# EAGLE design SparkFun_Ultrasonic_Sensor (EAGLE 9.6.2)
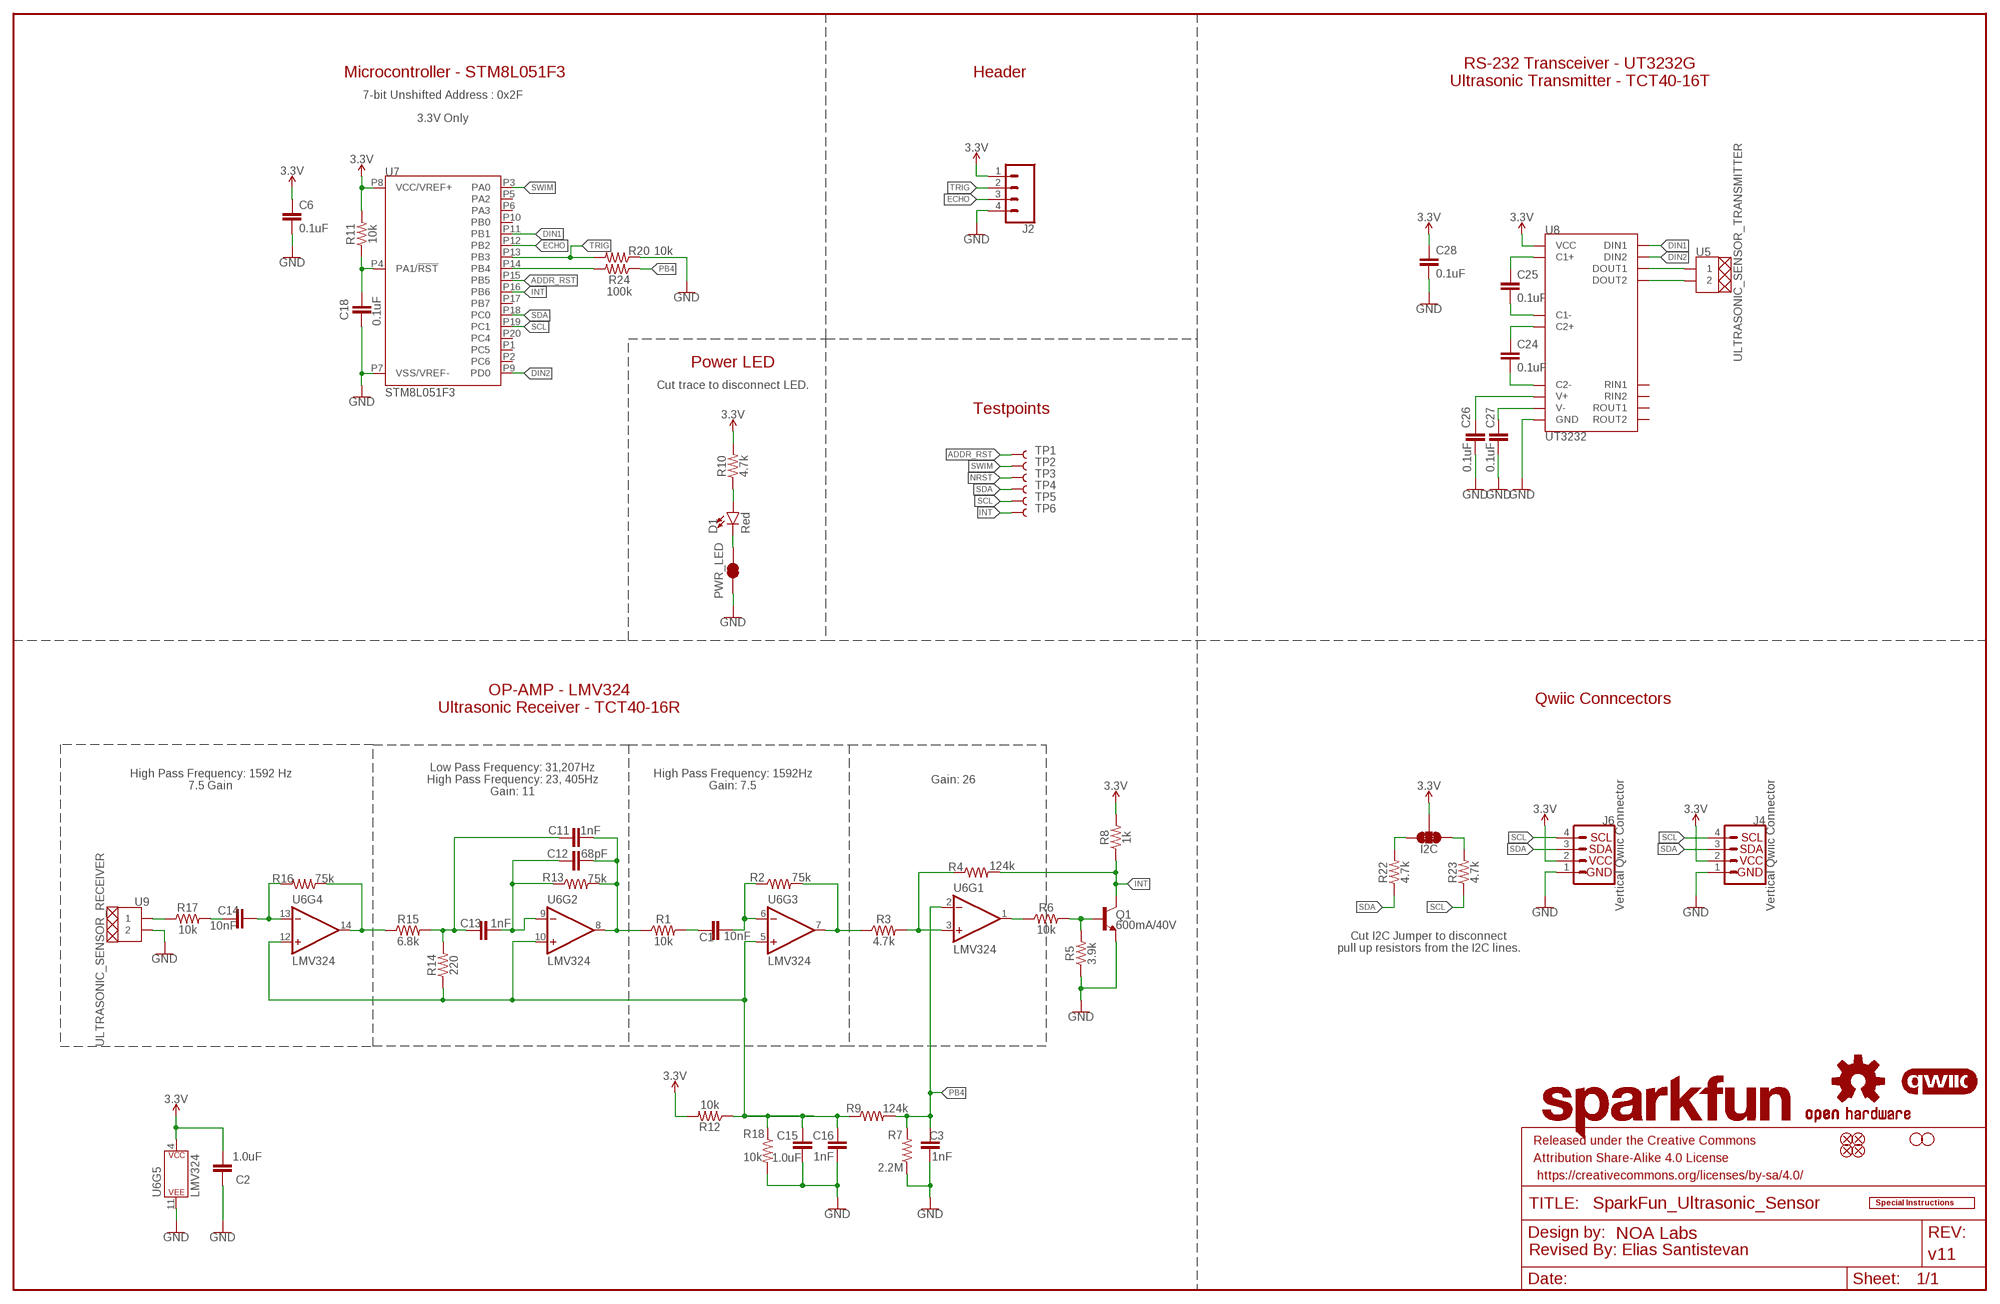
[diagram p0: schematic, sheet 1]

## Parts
C1  10nF  10NF-0603-50V-10%  [0603]
C2  1.0uF  1.0UF-0603-16V-10%  [0603]
C3  1nF  1.0NF/1000PF-0603-50V-10%  [0603]
C6  0.1uF  0.1UF-0603-25V-(+80/-20%)  [0603]
C11  1nF  1.0NF/1000PF-0603-50V-10%  [0603]
C12  68pF  68PF-0603-50V-5%  [0603]
C13  1nF  1.0NF/1000PF-0603-50V-10%  [0603]
C14  10nF  10NF-0603-50V-10%  [0603]
C15  1.0uF  1.0UF-0603-16V-10%  [0603]
C16  1nF  1.0NF/1000PF-0603-50V-10%  [0603]
C18  0.1uF  0.1UF-0603-25V-(+80/-20%)  [0603]
C24  0.1uF  0.1UF-0603-25V-(+80/-20%)  [0603]
C25  0.1uF  0.1UF-0603-25V-(+80/-20%)  [0603]
C26  0.1uF  0.1UF-0603-25V-(+80/-20%)  [0603]
C27  0.1uF  0.1UF-0603-25V-(+80/-20%)  [0603]
C28  0.1uF  0.1UF-0603-25V-(+80/-20%)  [0603]
D1  Red  LED-RED_0603-KB  [LED-0603]
FD1  FIDUCIAL1X2  [FIDUCIAL-1X2]
FD2  FIDUCIAL1X2  [FIDUCIAL-1X2]
FD3  FIDUCIAL1X2  [FIDUCIAL-1X2]
FD4  FIDUCIAL1X2  [FIDUCIAL-1X2]
FRAME1  FRAME-LEDGER  [CREATIVE_COMMONS]
H1  STAND-OFFTIGHT  [STAND-OFF-TIGHT]
H2  STAND-OFFTIGHT  [STAND-OFF-TIGHT]
I2C  JUMPER-SMT_3_2-NC_TRACE_SILK  [SMT-JUMPER_3_2-NC_TRACE_SILK]
J2  CONN_041X04_NO_SILK_NO_POP  [1X04_NO_SILK]
J4  Vertical Qwiic Connector  QWIIC_CONNECTOR  [JST04_1MM_VERT]
J6  Vertical Qwiic Connector  QWIIC_CONNECTOR  [JST04_1MM_VERT]
LOGO1  SPECIAL_INSTRUCTIONS-ORDERING  [ORDERING_INSTRUCTIONS]
LOGO2  SFE_LOGO_NAME.1_INCH  [SFE_LOGO_NAME_.1]
LOGO3  QWIIC_LOGO_3MM  [QWIIC_3MM]
LOGO4  OSHW-LOGOS  [OSHW-LOGO-S]
PWR_LED  JUMPER-SMT_2_NC_TRACE_SILK  [SMT-JUMPER_2_NC_TRACE_SILK]
Q1  600mA/40V  TRANS_NPN-MMBT2222AL  [SOT23-3]
R1  10k  10KOHM-0603-1/10W-1%  [0603]
R2  75k  75KOHM-0603-1/10W-1%  [0603]
R3  4.7k  4.7KOHM-0603-1/10W-1%  [0603]
R4  124k  124KOHM  [0603]
R5  3.9k  3.9KOHM-0603-1/10W-1%  [0603]
R6  10k  10KOHM-0603-1/10W-1%  [0603]
R7  2.2M  2.2MOHMS-0603-1/10W-1%  [0603]
R8  1k  1KOHM-0603-1/10W-1%  [0603]
R9  124k  124KOHM  [0603]
R10  4.7k  4.7KOHM-0603-1/10W-1%  [0603]
R11  10k  10KOHM-0603-1/10W-1%  [0603]
R12  10k  10KOHM-0603-1/10W-1%  [0603]
R13  75k  75KOHM-0603-1/10W-1%  [0603]
R14  220  220OHM-0603-1/10W-1%  [0603]
R15  6.8k  6.8KOHM-0603-1/10W-1%  [0603]
R16  75k  75KOHM-0603-1/10W-1%  [0603]
R17  10k  10KOHM-0603-1/10W-1%  [0603]
R18  10k  10KOHM-0603-1/10W-1%  [0603]
R20  10k  10KOHM-0603-1/10W-1%  [0603]
R22  4.7k  4.7KOHM-0603-1/10W-1%  [0603]
R23  4.7k  4.7KOHM-0603-1/10W-1%  [0603]
R24  100k  100KOHM-0603-1/10W-1%  [0603]
TP1  TEST-POINT3X5  [PAD.03X.05]
TP2  TEST-POINT3X5  [PAD.03X.05]
TP3  TEST-POINT3X5  [PAD.03X.05]
TP4  TEST-POINT3X5  [PAD.03X.05]
TP5  TEST-POINT3X5  [PAD.03X.05]
TP6  TEST-POINT3X5  [PAD.03X.05]
U5  ULTRASONIC_SENSOR_TRANSMITTER  [TFT40-16T]
U6  LMV324  [SO14]
U7  STM8L051F3  [TSSOP20]
U8  UT3232  [TSSOP16]
U9  ULTRASONIC_SENSOR_RECEIVER  [TCT40-16R]

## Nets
3.3V: C2.2 C6.1 C28.1 I2C.2 J2.1 J4.2 J6.2 R8.2 R10.2 R11.2 R12.2 U6.4(P$V+) U7.P8(VCC/VREF+) U8.P16(VCC)
ADDR_RST: TP1.1 U7.P15(PB5)
DIN1: U7.P11(PB1) U8.P11(DIN1)
DIN2: U7.P9(PD0) U8.P10(DIN2)
ECHO: J2.3 U7.P12(PB2)
GND: C2.1 C3.2 C6.2 C15.1 C16.1 C18.2 C26.2 C27.2 C28.2 J2.4 J4.1 J6.1 PWR_LED.1 Q1.2(E) R5.1 R7.1 R18.2 R20.1 U6.11(P$V-) U7.P7(VSS/VREF-) U8.P15(GND) U9.P2
INT: Q1.3(C) R4.2 R8.1 TP6.1 U7.P16(PB6)
N: R24.2 U7.P14(PB4)
N$1: R2.2 R3.1 U6.7(OUT)
N$2: C1.1 R2.1 U6.6(-IN)
N$3: C1.2 R1.2
N$4: R3.2 R4.1 U6.3(+IN)
N$5: Q1.1(B) R5.2 R6.2
N$6: R6.1 U6.1(OUT)
N$7: D1.A R10.1
N$8: C25.1 U8.P1(C1+)
N$9: C12.1 C13.1 R13.1 U6.9(-IN)
N$10: C11.2 C12.2 R1.1 R13.2 U6.8(OUT)
N$11: D1.C PWR_LED.2
N$12: C11.1 C13.2 R14.2 R15.2
N$14: R15.1 R16.1 U6.14(OUT)
N$15: C14.1 R16.2 U6.13(-IN)
N$16: C14.2 R17.2
N$19: I2C.3 R22.2
N$20: I2C.1 R23.2
N$26: R17.1 U9.P1
N$31: C15.2 C16.2 R9.1 R12.1 R14.1 R18.1 U6.5(+IN) U6.10(+IN) U6.12(+IN)
N$37: C25.2 U8.P3(C1-)
N$38: C24.1 U8.P4(C2+)
N$39: C24.2 U8.P5(C2-)
N$40: C27.1 U8.P6(V-)
N$41: C26.1 U8.P2(V+)
N$48: U5.P1 U8.P14(DOUT1)
N$49: U5.P2 U8.P7(DOUT2)
NRST: C18.1 R11.1 TP3.1 U7.P4(PA1/!RST!)
PB4: C3.1 R7.2 R9.2 R24.1 U6.2(-IN)
SCL: J4.4 J6.4 R23.1 TP5.1 U7.P19(PC1)
SDA: J4.3 J6.3 R22.1 TP4.1 U7.P18(PC0)
SWIM: TP2.1 U7.P3(PA0)
TRIG: J2.2 R20.2 U7.P13(PB3)
Unconnected: U7.P1(PC5) U7.P2(PC6) U7.P5(PA2) U7.P6(PA3) U7.P10(PB0) U7.P17(PB7) U7.P20(PC4) U8.P8(RIN2) U8.P9(ROUT2) U8.P12(ROUT1) U8.P13(RIN1)

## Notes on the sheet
- Microcontroller - STM8L051F3 | Header
- RS-232 Transceiver - UT3232G
  Ultrasonic Transmitter - TCT40-16T
- 7-bit Unshifted Address : 0x2F
- 3.3V Only
- Power LED
- Cut trace to disconnect LED.
- Testpoints
- OP-AMP - LMV324
  Ultrasonic Receiver - TCT40-16R
- Qwiic Conncectors
- High Pass Frequency: 1592 Hz
  7.5 Gain
- Low Pass Frequency: 31,207Hz
  High Pass Frequency: 23, 405Hz
  Gain: 11
- High Pass Frequency: 1592Hz
  Gain: 7.5
- Gain: 26
- Cut I2C Jumper to disconnect
  pull up resistors from the I2C lines.
- Revised By: Elias Santistevan

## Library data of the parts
C1 C14 = SparkFun-Capacitors:10NF: 0.01uF/10nF/10,000pF ceramic capacitors; PROD_ID: CAP-00867
C2 C15 = SparkFun-Capacitors:1.0UF: 1µF ceramic capacitors; PROD_ID: CAP-00868
C3 C11 C13 C16 = SparkFun-Capacitors:1.0NF/1000PF: 1nF/1,000pF ceramic capacitors; PROD_ID: CAP-07886
C6 C18 C24-C28 = SparkFun-Capacitors:0.1UF: 0.1µF ceramic capacitors; PROD_ID: CAP-00810
C12 = SparkFun-Capacitors:68PF: 68pF ceramic capacitors; PROD_ID: CAP-14092
D1 = SparkFun-LED:LED-RED: Red SMD LED; PROD_ID: DIO-17976
FD1-FD4 = SparkFun-Aesthetics:FIDUCIAL: Fiducial Alignment Points
FRAME1 = SparkFun-Aesthetics:FRAME-LEDGER: Schematic Frame - Ledger; DESIGNER: NOA Labs; REV: v11
H1 H2 = SparkFun-Hardware:STAND-OFF: Stand Off
I2C = SparkFun-Jumpers:JUMPER-SMT_3_2-NC_TRACE: Normally closed trace jumper (2 of 2 connections) This jumper has a trace between all three pads so they are normally closed (NC). Use a razor knife to open the connection(s). For best results follow the IPC guidelines for cutting traces: Cutout at least 0.063 mm (0.005 in). Remove all loose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
J2 = SparkFun-Connectors:CONN_04: Multi connection point. Often used as Generic Header-pin footprint for 0.1 inch spaced/style header connections On any of the 0.1 inch spaced packages, you can populate with these: Break Away Headers - Straight (PRT-00116) Break Away Male Headers - Right Angle (PRT-00553) Female Headers (PRT-00115)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
J4 J6 = SparkFun-Connectors:QWIIC_CONNECTOR: SparkFun I2C Standard Qwiic Connector An SMD 1mm pitch JST connector makes it easy and quick (get it? Qwiic?) to connect I2C devices to each other. The Qwiic system enables fast and solderless connection between popular platforms and various sensors and actuators. We carry 200mm, 100mm, 50mm, and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; PROD_ID: CONN-14483
LOGO1 = SparkFun-Aesthetics:SPECIAL_INSTRUCTIONS: Special Ordering/Production Instructions Alert
LOGO2 = SparkFun-Aesthetics:SFE_LOGO_NAME: SparkFun Font Logo
LOGO3 = SparkFun-Aesthetics:QWIIC_LOGO: Qwiic Logos for placement on schematic and PCB. The 5.5mm silk logo is best for placing next to Qwiic connector.
LOGO4 = SparkFun-Aesthetics:OSHW-LOGO: Open-Source Hardware (OSHW) Logo
PWR_LED = SparkFun-Jumpers:JUMPER-SMT_2_NC_TRACE: Normally closed trace jumper
Q1 = SparkFun-DiscreteSemi:TRANS_NPN: NPN transistor Current controlled devices typically used to amplify current or used as a switch. BC547 - COM-08928 (TO-92 45V 100mA) (1.Collector 2.Base 3.Emitter) 2N3904 - COM-00521 (TO-92 40V 200mA) (1.Emitter 2.Base 3.Collector) P2N2222A - COM-12852 (TO-92 40V 600mA) (1.Collector 2.Base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; PROD_ID: TRANS-08049
R1 R6 R11 R12 R17 R18 R20 = SparkFun-Resistors:10KOHM: 10kΩ resistor; PROD_ID: RES-00824
R2 R13 R16 = SparkFun-Resistors:75KOHM: 75kΩ resistor; PROD_ID: RES-09737
R3 R10 R22 R23 = SparkFun-Resistors:4.7KOHM: 4.7kΩ resistor; PROD_ID: RES-07857
R4 R9 = SparkFun-Resistors:124KOHM: 124kΩ resistor; PROD_ID: RES-14395
R5 = SparkFun-Resistors:3.9KOHM: 3.9kΩ resistor; PROD_ID: RES-08701
R7 = SparkFun-Resistors:2.2MOHMS: 2MΩ resistor; PROD_ID: RES-10054
R8 = SparkFun-Resistors:1KOHM: 1kΩ resistor; PROD_ID: RES-07856
R14 = SparkFun-Resistors:220OHM: 220Ω resistor; PROD_ID: RES-07861
R15 = SparkFun-Resistors:6.8KOHM: 6.8kΩ resistor; PROD_ID: RES-08597
R24 = SparkFun-Resistors:100KOHM: 100kΩ resistor; PROD_ID: RES-07828
TP1-TP6 = SparkFun-Connectors:TEST-POINT: SparkFun Test Points
U5 = new_parts:ULTRASONIC_SENSOR: CU Devices - CUSA-R/T80; PROD_ID: SEN-21316
U6 = SparkFun-IC-Amplifiers:LMV324: IC LMV324 Quad Op Amp Jellybean quad op-amp Datasheet SparkFun Products SparkFun Sensor Kit (DEV-13754) SparkFun Inventor's Kit for Arduino 101 (KIT-13844) SparkFun Sound Detector (SEN-12642); PROD_ID: IC-08227
U7 = new_parts:STM8L051F3: ST STM8L051F3 Low-Power MCU STM8L051F3 features an enhanced STM8 CPU core providing increased processing power (up to 16 MIPS at 16 MHz) while maintaining the advantages of a CISC architecture with improved code density, a 24-bit linear addressing space and an optimized architecture for low-power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; PROD_ID: IC-21318
U8 = new_parts:UT3232: Unisonic Technologies - UT3232 TThe UTC UT3232 has two receivers and two drivers, and a dual charge-pump circuit. The device meets the requirements of TIA/EIA-232-F and provides the electrical interface between an asynchronous communication controller and the serial-port connector. The charge pump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; PROD_ID: IC-21317
U9 = new_parts:ULTRASONIC_SENSOR: CU Devices - CUSA-R/T80; PROD_ID: SEN-21315

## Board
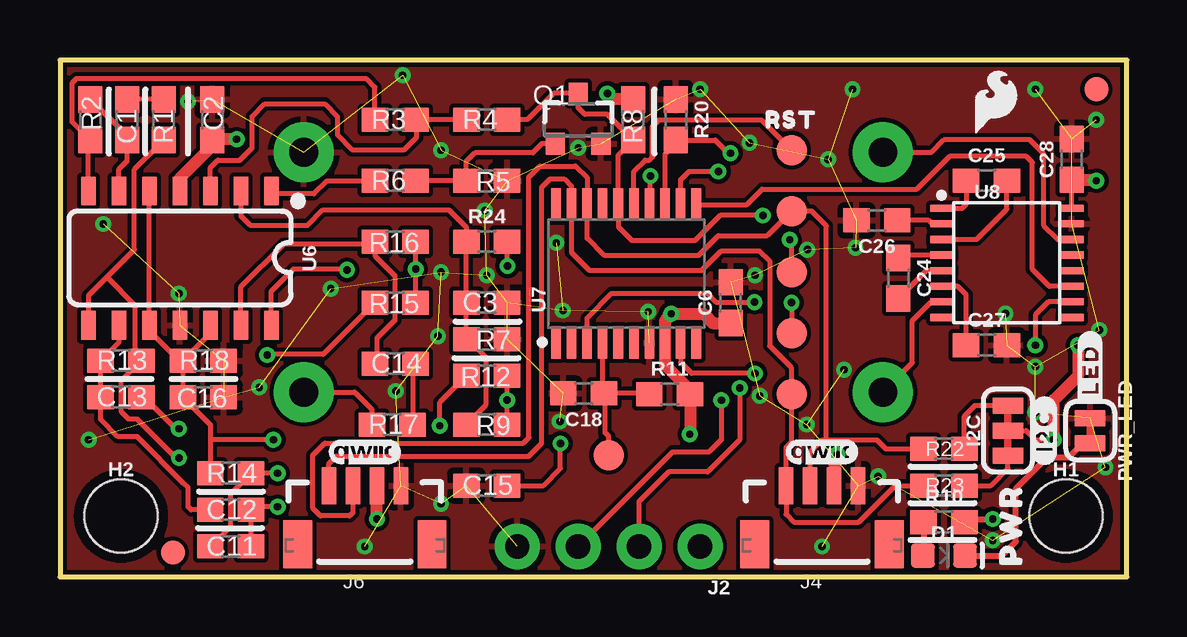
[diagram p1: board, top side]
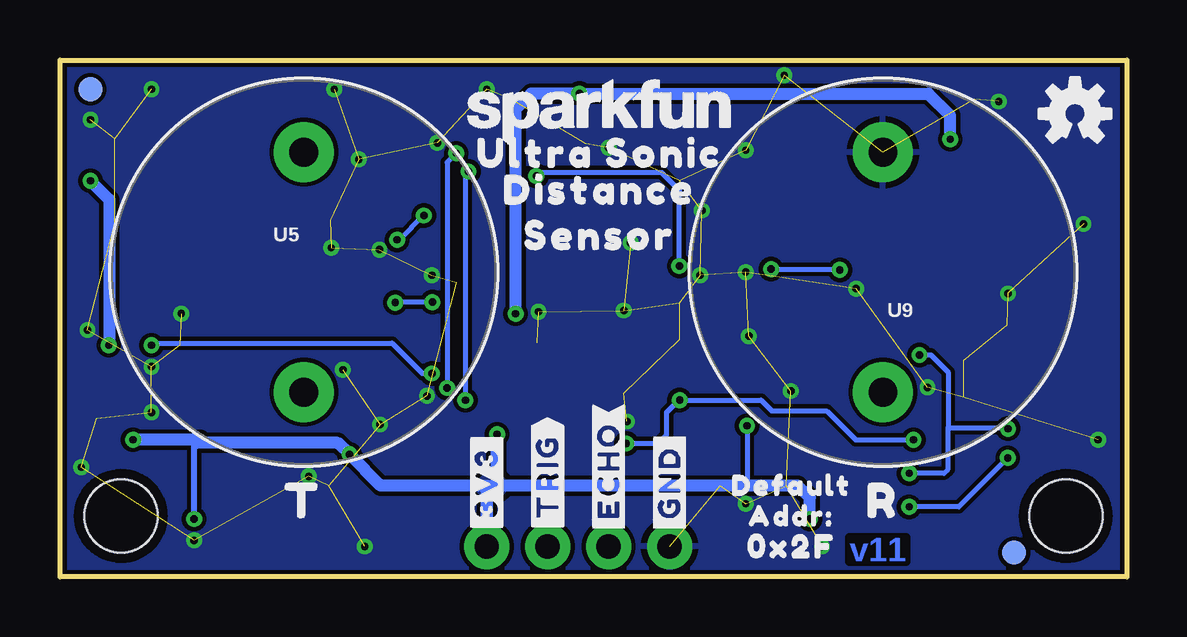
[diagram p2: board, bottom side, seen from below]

Size 44.45 x 21.54 mm. Coordinates in mm from the lower left corner, seen from the top.
Outline: 0,0 44.45,0 44.45,21.54 0,21.54 0,0
Copper layers (1+16): Top 0.035559375mm / dielectric 0.47751875mm / Bottom 0.035559375mm
Design rules "SparkFun-4-Layer-General-JLCPCB *": minimum track width 7mil, minimum drill 12mil, track to track 7mil, track to pad 7mil, pad to pad 7mil, via to via 7mil, smd to smd 7mil, copper to edge 7mil, drill to drill 7mil, minimum pad ring 7mil, minimum via ring 7mil, stop-mask expansion 3mil, vias tented up to drill 25mil, thermal gap 10mil

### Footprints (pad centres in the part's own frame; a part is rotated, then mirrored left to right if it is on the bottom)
0603 = smd 1.1 x 1: 1 -0.85,0; 2 0.85,0
LED-0603 = smd 1 x 1: A -0.877,0; C 0.877,0
FIDUCIAL-1X2 = smd 1 x 1: 1 0,0
STAND-OFF-TIGHT = hole 3.048: 0,0
SMT-JUMPER_3_2-NC_TRACE_SILK = smd 0.66 x 1.27: 1 -1.041,0; 2 0,0; 3 1.041,0
1X04_NO_SILK = drill 1.016 pad 1.88: 1 0,0; 2 2.54,0; 3 5.08,0; 4 7.62,0
JST04_1MM_VERT = smd 0.6 x 1.55: 1 -1.5,0.775; 2 -0.5,0.775; 3 0.5,0.775; 4 1.5,0.775 | smd 1.2 x 2: NC1 -2.8,3.2; NC2 2.8,3.2
SMT-JUMPER_2_NC_TRACE_SILK = smd 0.66 x 1.27: 1 -0.521,0; 2 0.521,0
SOT23-3 = smd 0.8 x 0.9: 1 -0.95,-1; 2 0.95,-1; 3 0,1.1
PAD.03X.05 = smd 1.27 x 1.27: 1 0,0
TFT40-16T = drill 1.2 pad 2.5: P1 0,5; P2 0,-5
SO14 = smd 0.6 x 1.2: 1 -3.175,-2.8; 2 -1.905,-2.8; 3 -0.635,-2.8; 4 0.635,-2.8; 5 1.905,-2.8; 6 3.175,-2.8; 7 4.445,-2.8; 8 4.445,2.8; 9 3.175,2.8; 10 1.905,2.8; 11 0.635,2.8; 12 -0.635,2.8; 13 -1.905,2.8; 14 -3.175,2.8
TSSOP20 = smd 1.35 x 0.4: P1 -2.911,2.878; P2 -2.911,2.228; P3 -2.911,1.578; P4 -2.911,0.928; P5 -2.911,0.278; P6 -2.911,-0.372; P7 -2.911,-1.022; P8 -2.911,-1.672; P9 -2.911,-2.322; P10 -2.911,-2.972; P11 2.839,-2.972; P12 2.839,-2.322; P13 2.839,-1.672; P14 2.839,-1.022; P15 2.839,-0.372; P16 2.839,0.278; P17 2.839,0.928; P18 2.839,1.578; P19 2.839,2.228; P20 2.839,2.878
TSSOP16 = smd 1 x 0.3: P1 -2.607,2.153; P2 -2.607,1.503; P3 -2.607,0.853; P4 -2.607,0.203; P5 -2.607,-0.447; P6 -2.607,-1.097; P7 -2.607,-1.747; P8 -2.607,-2.397; P9 2.793,-2.397; P10 2.793,-1.747; P11 2.793,-1.097; P12 2.793,-0.447; P13 2.793,0.203; P14 2.793,0.853; P15 2.793,1.503; P16 2.793,2.153
TCT40-16R = drill 1.2 pad 2.5: P1 0,5; P2 0,-5

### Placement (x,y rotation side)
C1  2.79,19.05 90 top
C2  6.35,19.05 270 top
C3  17.78,11.43 0 top
C6  27.94,11.43 90 top
C11  7.11,1.27 0 top
C12  7.11,2.79 0 top
C13  2.54,7.49 0 top
C14  13.97,8.89 0 top
C15  17.78,3.81 0 top
C16  5.97,7.49 180 top
C18  21.82,7.65 180 top
C24  34.92,12.45 270 top
C25  38.61,16.51 0 top
C26  34.04,14.86 180 top
C27  38.61,9.65 0 top
C28  42.16,17.4 90 top
D1  36.83,0.89 0 top
FD1  4.7,1.02 90 top
FD2  43.18,20.32 90 top
FD3  43.18,20.32 90 bottom
FD4  4.7,1.02 90 bottom
FRAME1  not placed on the board
H1  41.91,2.54 0 top
H2  2.54,2.54 0 top
I2C  39.5,6.1 90 top
J2  26.67,1.27 180 top
J4  31.75,4.57 180 top
J6  12.7,4.57 180 top
LOGO1  not placed on the board
LOGO2  21.97,19.3 0 bottom
LOGO3  12.7,5.21 0 top
LOGO4  2.16,19.3 0 bottom
PWR_LED  42.93,6.1 270 top
Q1  21.59,19.05 0 top
R1  4.32,19.05 90 top
R2  1.27,19.05 270 top
R3  13.97,19.05 0 top
R4  17.78,19.05 0 top
R5  17.78,16.51 180 top
R6  13.97,16.51 0 top
R7  17.78,9.91 180 top
R8  23.88,19.05 90 top
R9  17.78,6.35 180 top
R10  36.83,2.29 0 top
R11  25.4,7.62 0 top
R12  17.78,8.38 180 top
R13  2.54,9.02 0 top
R14  7.11,4.32 0 top
R15  13.97,11.43 180 top
R16  13.97,13.97 180 top
R17  13.84,6.35 0 top
R18  5.97,9.02 0 top
R20  25.65,19.05 270 top
R22  36.83,5.33 0 top
R23  36.83,3.81 0 top
R24  17.78,13.97 0 top
TP1  30.48,17.78 0 top
TP2  30.48,10.16 0 top
TP3  22.86,5.08 0 top
TP4  30.48,15.24 0 top
TP5  30.48,7.62 0 top
TP6  30.48,12.7 0 top
U5  34.29,12.7 0 bottom
U6  5.63,13.29 180 top
U7  23.54,12.68 90 top
U8  39.37,13.21 0 top
U9  10.16,12.7 180 bottom
U$1  [#ECHO#0]  21.59,4.45 90 bottom
U$2  [#TRIG#1]  24.13,4.19 90 bottom
U$3  [#GND#4]  19.05,3.94 90 bottom
U$4  [#3V3#2]  26.67,3.94 90 bottom
U$5  [QWIIC_3MM]  31.75,5.21 0 top
U$6  [SFE_LOGO_FLAME_.1]  38.99,19.81 0 top
U$7  [#I2C#16]  41.02,6.1 90 top
U$8  [T103]  34.29,3.17 0 bottom
U$9  [R104]  10.16,3.17 0 bottom
U$10  [DISTANCE101]  21.97,16.13 0 bottom
U$11  [ULTRA_SONIC100]  21.97,17.65 0 bottom
U$12  [SENSOR102]  21.97,14.22 0 bottom
U$13  [DEFAULT129]  13.97,3.81 0 bottom
U$14  [ADDR#130]  13.97,2.54 0 bottom
U$15  [0X2F131]  13.97,1.27 0 bottom
U$16  [PWR17]  39.62,2.16 90 top
U$17  [#LED#15]  42.93,8.64 90 top
U$18  [RST132]  30.48,19.05 0 top

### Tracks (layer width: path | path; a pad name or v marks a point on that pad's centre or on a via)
3.3V  (via drill 0.3)
  Top 0.203: U8.P16 C28.1 | I2C.2 40.26,6.1 40.64,5.71 v41.4,5.71 | R12.2 15.82,7.28 v15.82,6.3
  Top 0.254: R10.2 37.81,2.41 v38.86,2.41
  Top 0.508: v42.42,9.65 42.42,8.38 41.4,7.37 v41.4,5.71 | R8.2 23.05,19.9 v22.81,20.14 | v26.24,5.94 26.25,5.96 R11.2 26.25,7.79 25.21,8.82 U7.P8 25.21,10.67 25.27,10.73 25.27,10.77 v25.47,10.96 26.81,10.96 27.2,10.58 C6.1 | U6.4 5,16.6 6.35,17.96 C2.2 6.39,18.24 v7.36,18.24 | v32.38,5.11 32.25,4.97 J4.2 | C28.1 43.14,16.55 v43.18,16.51 | v13.21,2.41 13.2,2.42 J6.2
  Bottom 0.203: v15.82,6.3 15.82,3.89 15.75,3.81
  Bottom 0.254: v38.86,2.41 38.86,5.46 38.73,5.59 38.61,5.71
  Bottom 0.508: v42.42,9.65 42.39,9.68 42.39,15.72 v43.18,16.51 | v25.47,10.96 25.47,19.49 24.82,20.14 v22.81,20.14 8.27,20.14 7.36,19.23 v7.36,18.24 | 38.73,5.59 32.87,5.59 v32.38,5.11 31.09,3.81 26.67,3.81 J2.1 26.67,3.4 26.26,3.81 | 38.61,5.71 v41.4,5.71 | 26.26,3.81 15.75,3.81 13.72,3.81 13.21,3.3 v13.21,2.41 | v26.24,5.94 26.26,5.92 26.26,3.81
  pour Bottom (isolate 0.305, no thermals): 26.44,4.35 25.93,3.79 26.51,3.29 26.98,3.77
ADDR_RST
  Top 0.203: U7.P15 23.91,16.9 24.38,17.37 24.57,17.37 24.68,17.48 24.68,18.76 24.95,19.03 29.23,19.03 TP1.1
DIN1
  Top 0.203: U8.P11 41.23,12.11 40.51,12.83 40.51,17.27 40.26,17.53 37.08,17.53 35.7,16.15 29.26,16.15 28.62,15.52 U7.P11
DIN2  (via drill 0.3)
  Top 0.203: U8.P10 41.18,11.46 40.64,10.92 v40.64,9.65 | U7.P9 25.86,8.94 26.31,8.48 28.95,8.48 v28.96,8.47
  Bottom 0.203: v28.96,8.47 29.34,8.47 30.61,9.74 40.55,9.74 v40.64,9.65
ECHO  (via drill 0.3)
  Top 0.203: v27.43,16.89 26.2,16.89 25.86,16.55 U7.P12 | J2.3 25.53,5.21 27.05,5.21 27.56,5.71 v27.56,7.36
  Bottom 0.203: v27.43,16.89 27.56,16.76 v27.56,7.36
GND  (via drill 0.3)  (61 unrouted)
  other vias: 33.15,13.72 24.51,11.05 15.88,3.05 34.09,4.19 5.33,19.81 17.78,12.57 20.83,6.48 8.31,7.9 4.95,11.81 26.67,20.32 21.59,17.88 29.16,7.54 17.7,15.27 40.64,8.76 15.75,10.03 15.88,12.7 28.96,12.57 11.28,12.01 14,7.75 15.88,17.78 20.95,11.1 20.68,13.92 32,17.4 39.4,10.97 1.8,14.71 12.7,1.27 31.75,1.27 38.86,1.52 43.31,10.29 43.18,19.05 40.64,20.32 33.02,20.32 14.27,20.9 32.66,8.64 1.19,5.71 31.14,13.64 31.11,6.35 28.73,18.08 43.56,4.57 40.64,6.86
  pour Top (rank 3): 0,21.54 44.45,21.54 44.45,0 0,0
  pour Bottom (rank 4): 0,21.54 44.45,21.54 44.45,0 0,0
INT  (via drill 0.3)
  Top 0.203: R4.2 19.47,19.05 20.57,20.15 Q1.3 21.59,19.56 21.87,19.28 22.8,19.28 R8.1 23.26,17.59 U7.P16 23.26,14.58 23.82,14.02 26.47,14.02 27.53,15.09 29.26,15.09 v29.29,15.06 | TP6.1 30.48,13.97 v30.4,14.05
  Bottom 0.203: v30.4,14.05 30.3,14.05 v29.29,15.06
N  (via drill 0.3)
  Top 0.203: U7.P14 24.6,15.56 v24.6,16.7 | R24.2 18.63,12.97 v18.64,12.95
  Bottom 0.203: v18.64,12.95 18.64,16.1 19.4,16.86 24.45,16.86 v24.6,16.7
N$1
  Top 0.203: U6.7 1.19,18.11 R2.2 0.49,18.98 0.49,20.57 0.68,20.75 12.78,20.75 13.12,20.41 R3.1
N$2
  Top 0.203: U6.6 2.46,17 2.79,17.34 C1.1 2.79,18.38 R2.1
N$3
  Top 0.203: R1.2 C1.2
N$4
  Top 0.203: R4.1 R3.2 14.86,19.01 14.86,18.31 14.35,17.8 12.17,17.8 11.56,18.41 11.56,19.18 11.03,19.71 8.53,19.71 8,19.18 8,17.88 7.49,17.37 6.58,17.37 6.26,17.06 U6.3
N$5
  Top 0.203: R6.2 R5.2 16.93,17.31 17.29,17.67 19.7,17.67 20.08,18.05 Q1.1
N$6
  Top 0.203: U6.1 8.8,15.96 10.58,15.96 11.12,16.5 13.11,16.5 R6.1
N$7
  Top 0.254: R10.1 35.98,0.92 D1.A
N$8
  Top 0.203: U8.P1 37.59,15.36 37.76,15.53 C25.1
N$9
  Top 0.203: U6.9 2.46,9.78 R13.1 C13.1 1.69,6.57 2.41,5.84 3.21,5.84 5.16,3.89 5.33,3.72 5.33,2.92 5.46,2.79 C12.1
N$10  (via drill 0.3)
  Top 0.203: 1.97,12.51 3.1,13.64 3.1,16.98 R1.1 | 1.97,12.51 1.19,11.73 U6.8 | C11.2 C12.2 8.09,2.92 v9.07,2.92 | v4.96,4.96 4.82,4.96 3.19,6.59 2.85,6.59 2.56,6.88 2.56,8.2 3.38,9.02 R13.2 3.39,9.27 3.15,9.52 3.15,11.31 1.97,12.48 1.97,12.51
  Bottom 0.203: v4.96,4.96 7,2.92 v9.07,2.92
N$11
  Top 0.254: PWR_LED.2 42.62,5.58 42.02,4.98 41.14,4.98 39.83,3.67 39.83,1.47 39.24,0.89 D1.C
N$12  (via drill 0.3)
  Top 0.203: R15.2 10.96,9.27 8.89,9.27 8.87,9.25 v8.64,9.25 | C11.1 7.11,2.12 7.11,3.47 R14.2 v9.07,4.32 | C13.2 3.51,7.49 4.83,6.18 v4.95,6.18
  Bottom 0.203: v8.64,9.25 8.16,9.25 7.44,8.53 7.44,6.22 | v9.07,4.32 7.62,4.32 7.44,4.5 7.44,6.22 | 7.44,6.22 5,6.22 v4.95,6.18
N$14  (via drill 0.3)
  Top 0.203: U6.14 8.8,11.9 9.72,12.82 11.93,12.82 v11.96,12.79 | R15.1 v14.82,12.83 R16.1
  Bottom 0.203: v14.82,12.83 11.99,12.83 v11.96,12.79
N$15
  Top 0.203: C14.1 13.21,8.98 13.21,9.95 13.95,10.69 13.95,12.55 13.12,13.38 R16.2 13.02,13.87 9.32,13.87 7.54,12.08 U6.13
N$16
  Top 0.203: C14.2 14.69,8.76 R17.2
N$19
  Top 0.203: R22.2 37.68,6.71 38.11,7.14 I2C.3
N$20
  Top 0.203: R23.2 38.79,3.81 39.5,4.52 I2C.1
N$26
  Top 0.203: R17.1 12.99,6.99 12.28,7.7 U9.P1
N$31  (via drill 0.3)
  Top 0.203: R18.1 C16.2 6.26,6.35 6.26,5.71 | U6.12 6.26,10.16 R18.1 | U6.5 U6.10 3.73,10.25 4.96,9.02 R18.1 | C15.2 20.14,3.81 20.85,4.52 v20.85,5.56 | R12.1 v18.63,7.37 R9.1 | 6.26,5.71 R14.1 | v8.89,5.71 6.26,5.71
  Bottom 0.203: v20.85,5.56 19.53,5.56 19.18,5.92 19.18,6.86 18.67,7.37 v18.63,7.37 15.24,7.37 14.8,6.92 12.51,6.92 11.3,5.71 v8.89,5.71
N$37
  Top 0.203: C25.2 39.46,15.33 38.19,14.06 U8.P3
N$38
  Top 0.203: U8.P4 35.04,13.41 C24.1
N$39
  Top 0.203: U8.P5 36.09,12.76 C24.2
N$40
  Top 0.203: C27.1 37.76,11.77 37.41,12.11 U8.P6
N$41
  Top 0.203: U8.P2 36.34,14.71 36.2,14.86 C26.1
N$48
  Top 0.203: U8.P14 41.56,14.06 40.97,14.66 40.97,17.65 40.41,18.21 36.83,18.21 36.32,17.7 U5.P1
N$49
  Top 0.203: U8.P7 36.3,11.46 35.52,10.68 35.52,8.93 U5.P2
NRST
  Top 0.203: 22.65,7.63 C18.1 24.52,7.64 R11.1 | U7.P4 22.61,7.67 22.65,7.63 | TP3.1 22.86,5.87 22.71,6.02 22.71,7.57 22.65,7.63
PB4
  Top 0.203: U6.2 7.54,15.04 7.93,14.65 10.31,14.65 10.96,15.29 16.2,15.29 16.93,14.57 R24.1 C3.1 R7.2 16.98,9.91 17.76,9.12 17.76,7.18 R9.2
SCL
  Top 0.203: R23.1 34.8,3.81 33.27,2.29 30.57,2.29 30.25,2.61 J4.4 30.25,5.4 30.48,5.63 TP5.1 30.48,8.71 29.57,9.63 29.57,13.17 29.14,13.59 27.56,13.59 26.75,12.78 22.06,12.78 21.31,13.53 U7.P19 21.31,16.28 21.01,16.59 20.42,16.59 20.07,16.23 20.07,5.56 19.53,5.03 11.51,5.03 11.2,4.72 J6.4
SDA
  Top 0.203: 31.93,5.71 31.93,14.63 31.32,15.24 TP4.1 29.46,14.22 27.43,14.22 26.62,13.41 22.66,13.41 21.96,14.11 U7.P18 21.96,16.65 21.49,17.12 19.99,17.12 19.53,16.66 19.53,5.81 19.3,5.57 11.03,5.57 10.54,5.08 10.54,2.85 10.85,2.54 12.06,2.54 12.2,2.67 J6.3 | J4.3 31.25,5.21 31.75,5.71 31.93,5.71 | 31.93,5.71 34.03,5.71 34.42,5.33 R22.1
SWIM  (via drill 0.3)
  Top 0.203: U7.P3 21.96,10.79 22.99,11.81 26.96,11.81 27.32,11.45 v28.93,11.45 | v30.48,11.43 TP2.1
  Bottom 0.203: v28.93,11.45 30.46,11.45 v30.48,11.43
TRIG  (via drill 0.3)
  Top 0.203: U7.P13 25.21,17.63 25.65,18.07 R20.2 27.3,18.2 27.85,17.65 v27.94,17.65 | J2.2 24.13,3.15 25.36,4.38 26.99,4.38 28.32,5.71 v28.32,7.87
  Bottom 0.203: v27.94,17.65 28.32,17.27 v28.32,7.87

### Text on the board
Bottom: v11
Measures: Units In Inches
tDocu: Two Layer / 1.6mm Thickness / 1 oz. Copper / Red Soldermask / White Silkscreen / HASL Lead Free / Material: TG135-140 | NOA Labs | Revised By: Elias Santistevan

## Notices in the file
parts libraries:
SparkFun-PowerSymbols: Licensing: Creative Commons ShareAlike 4.0 International - https://creativecommons.org/licenses/by-sa/4.0
SparkFun-Aesthetics: Released under the Creative Commons Attribution Share-Alike 4.0 License
SparkFun-Aesthetics: https://creativecommons.org/licenses/by-sa/4.0
